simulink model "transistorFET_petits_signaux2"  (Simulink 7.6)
settings: Solver=ode15s  StartTime=0.0  StopTime=0.06  RelTol=1e-3
InitFcn:
  | rho=1e6;
  | RD=1000;
  | RB1=47e3;
  | RB2=47e3;
  | RB=RB1*RB2/(RB1+RB2);
  | g=3000e-6;
StopFcn:
  | close all
  | load es.mat
  | plot(es(1,:),es(2,:),es(1,:),es(3,:))
  | title('Signaux d''E/S - Schéma équivalent du transistor FET')
  | xlabel('temps')
  | grid
libraries: fl_lib x9, nesl_utility x3

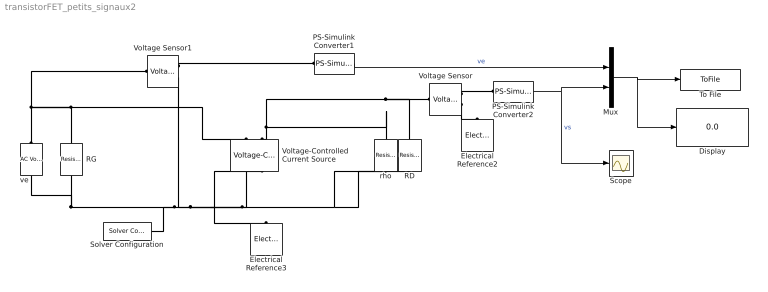
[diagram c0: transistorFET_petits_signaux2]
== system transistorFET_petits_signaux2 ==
  Display : Display
  Electrical Reference2 : fl_lib/Electrical/Electrical Elements/Electrical Reference  DialogController=NetworkEngine.DynNeDlgSource  SystemSampleTime=-1  i_Log=off  LocalVarNames=|i  LocalVarDescs=|i  LocalVarLogging=0
  Electrical Reference3 : fl_lib/Electrical/Electrical Elements/Electrical Reference  DialogController=NetworkEngine.DynNeDlgSource  SystemSampleTime=-1  i_Log=off  LocalVarNames=|i  LocalVarDescs=|i  LocalVarLogging=0
  Mux : Mux  Inputs=2
  PS-Simulink Converter1 : nesl_utility/PS-Simulink Converter  DialogController=NetworkEngine.DynNeUtilDlgSource  SystemSampleTime=-1  PhysicalDomain=network_engine_domain  LeftPortType=input  RightPortType=output  SubClassName=ps_output  Unit=1  AffineConversion=off
  PS-Simulink Converter2 : nesl_utility/PS-Simulink Converter  DialogController=NetworkEngine.DynNeUtilDlgSource  SystemSampleTime=-1  PhysicalDomain=network_engine_domain  LeftPortType=input  RightPortType=output  SubClassName=ps_output  Unit=1  AffineConversion=off
  RD : fl_lib/Electrical/Electrical Elements/Resistor  DialogController=NetworkEngine.DynNeDlgSource  SystemSampleTime=-1  R=RD Ohm  i_Log=off  v_Log=off  LocalVarNames=|i|v  LocalVarDescs=|i|v  LocalVarLogging=[0 0]
  RG : fl_lib/Electrical/Electrical Elements/Resistor  DialogController=NetworkEngine.DynNeDlgSource  SystemSampleTime=-1  R=rho Ohm  i_Log=off  v_Log=off  LocalVarNames=|i|v  LocalVarDescs=|i|v  LocalVarLogging=[0 0]
  Scope : Scope
  Solver Configuration : nesl_utility/Solver Configuration  DialogController=NetworkEngine.DynNeUtilDlgSource  SystemSampleTime=-1  PhysicalDomain=network_engine_domain  LeftPortType=input  RightPortType=generic  SubClassName=solver  Accelerate=off  Profile=off  ResidualTolerance=1e-9  MaxNonlinIter=3  MaxModeIter=2  DoFixedCost=off  UseLocalSampling=off  DoDC=off  LinearAlgebra=Sparse  LocalSolverSampleTime=.001  LocalSolverChoice=NE_BACKWARD_EULER_ADVANCER  UseLocalSolver=off
  To File : ToFile  Filename=es.mat  MatrixName=es
  Voltage Sensor : fl_lib/Electrical/Electrical Sensors/Voltage Sensor  DialogController=NetworkEngine.DynNeDlgSource  SystemSampleTime=-1  i1_Log=off  v1_Log=off  LocalVarNames=|i1|v1  LocalVarDescs=|i1|v1  LocalVarLogging=[0 0]
  Voltage Sensor1 : fl_lib/Electrical/Electrical Sensors/Voltage Sensor  DialogController=NetworkEngine.DynNeDlgSource  SystemSampleTime=-1  i1_Log=off  v1_Log=off  LocalVarNames=|i1|v1  LocalVarDescs=|i1|v1  LocalVarLogging=[0 0]
  Voltage-Controlled Current Source : fl_lib/Electrical/Electrical Sources/Voltage-Controlled Current Source  DialogController=NetworkEngine.DynNeDlgSource  SystemSampleTime=-1  K=-g 1/Ohm  i1_Log=off  v1_Log=off  i2_Log=off  v2_Log=off  LocalVarNames=|i1|v1|i2|v2  LocalVarDescs=|i1|v1|i2|v2  LocalVarLogging=[0 0 0 0]
  rho : fl_lib/Electrical/Electrical Elements/Resistor  DialogController=NetworkEngine.DynNeDlgSource  SystemSampleTime=-1  R=rho Ohm  i_Log=off  v_Log=off  LocalVarNames=|i|v  LocalVarDescs=|i|v  LocalVarLogging=[0 0]
  ve : fl_lib/Electrical/Electrical Sources/AC Voltage Source  DialogController=NetworkEngine.DynNeDlgSource  SystemSampleTime=-1  amp=10 mV  shift=0 rad  omega=60 Hz  i_Log=off  v_Log=off  LocalVarNames=|i|v  LocalVarDescs=|i|v  LocalVarLogging=[0 0]
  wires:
  PS-Simulink Converter2/1 -> Mux/2, Scope/1  "vs"
  PS-Simulink Converter1/1 -> Mux/1  "ve"
  Mux/1 -> To File/1, Display/1
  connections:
  RG/RConn1 -- Voltage-Controlled Current Source/LConn1 -- ve/LConn1 -- Voltage Sensor1/LConn1
  Voltage-Controlled Current Source/LConn2 -- RD/RConn1 -- Voltage Sensor/LConn1 -- rho/RConn1
  Voltage Sensor/RConn2 -- Electrical Reference2/LConn1
  Voltage Sensor/RConn1 -- PS-Simulink Converter2/LConn1
  Voltage-Controlled Current Source/RConn1 -- rho/LConn1 -- RD/LConn1 -- Voltage-Controlled Current Source/RConn2 -- Electrical Reference3/LConn1 -- RG/LConn1 -- ve/RConn1 -- Solver Configuration/RConn1 -- Voltage Sensor1/RConn2
  Voltage Sensor1/RConn1 -- PS-Simulink Converter1/LConn1
